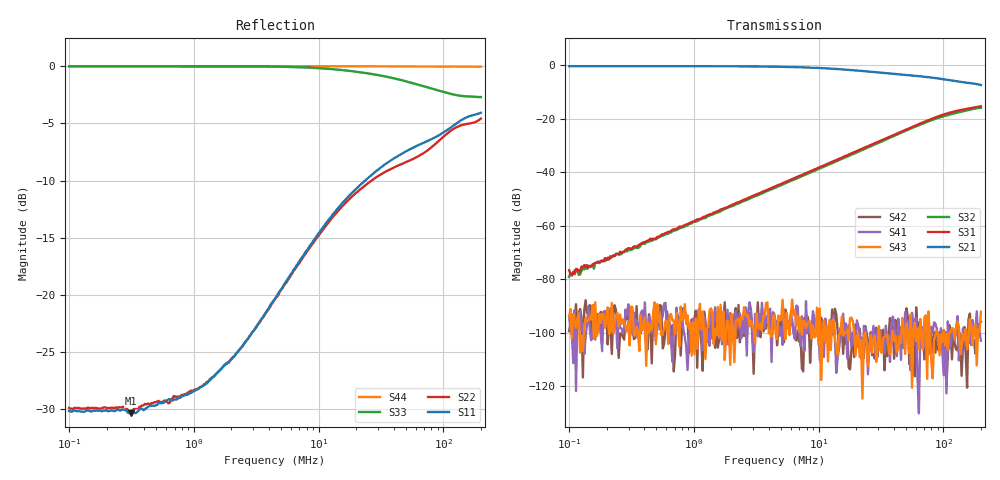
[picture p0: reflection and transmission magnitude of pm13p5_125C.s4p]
!Keysight Technologies,E5080A,MY55200740,A.12.60.03
!Date: Friday, October 02, 2020 16:46:49
!Correction: S11(Full 4 Port(1,2,3,4))
!S12(Full 4 Port(1,2,3,4))
!S13(Full 4 Port(1,2,3,4))
!S14(Full 4 Port(1,2,3,4))
!S21(Full 4 Port(1,2,3,4))
!S22(Full 4 Port(1,2,3,4))
!S23(Full 4 Port(1,2,3,4))
!S24(Full 4 Port(1,2,3,4))
!S31(Full 4 Port(1,2,3,4))
!S32(Full 4 Port(1,2,3,4))
!S33(Full 4 Port(1,2,3,4))
!S34(Full 4 Port(1,2,3,4))
!S41(Full 4 Port(1,2,3,4))
!S42(Full 4 Port(1,2,3,4))
!S43(Full 4 Port(1,2,3,4))
!S44(Full 4 Port(1,2,3,4))
!S4P File: Measurements: <S11,S12,S13,S14>,
!<S21,S22,S23,S24>,
!<S31,S32,S33,S34>,
!<S41,S42,S43,S44>:Log Frequency Sweep
# Hz S  dB  R 50
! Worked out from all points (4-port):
!   300 points, 100 kHz to 200 MHz, reference 50 ohm
!   strongest paths, dB at 100 kHz, 673 kHz, 4.529 MHz, 30.48 MHz, 200 MHz:
!     S21: -0.3, -0.3, -0.5, -2.6, -7.3
!     S31: -76.7, -61.5, -45.2, -28.4, -15.3
!     S32: -79.2, -62.0, -45.7, -28.9, -15.8
!     S43: -94.1, -95.5, -100.3, -97.6, -92.3
!     S41: -93.9, -111.0, -96.1, -104.5, -103.1
!     S42: -99.5, -97.3, -95.8, -100.9, -95.9
!   lowest |S11| = -30.3 dB at 313.9 kHz (marker M1), VSWR 1.06, Z = 53.1 - j0.415 ohm
!   |S11| at or under -10 dB: start of sweep to 23.56 MHz
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100000  -30.14 0.8  -0.28 -0.2  -77.77 103.0  -90.92 60.2
        -0.28 -0.1  -29.86 1.1  -78.88 67.9  -85.22 -115.2
        -76.69 78.8  -79.15 95.1  0.00 -0.1  -95.41 -79.3
        -93.87 -113.2  -99.46 -33.6  -94.12 -60.1  0.00 -0.0
105215.7  -30.20 0.5  -0.28 -0.2  -77.80 83.2  -103.98 -155.2
          -0.28 -0.1  -29.93 0.4  -80.37 91.0  -96.15 -156.7
          -78.67 102.4  -78.51 85.9  0.00 -0.1  -101.36 73.9
          -100.97 114.8  -98.27 -113.1  -102.19 69.2  0.00 -0.0
313913.9  -30.34 -7.4  -0.28 -0.4  -68.51 89.4  -97.13 -67.5
          -0.28 -0.4  -30.13 -7.3  -68.75 92.7  -117.84 -154.3
          -68.65 89.8  -69.02 84.8  0.00 -0.4  -93.11 13.3
          -92.06 -106.5  -98.51 -102.1  -90.35 37.1  0.00 -0.0
1908390  -25.91 -59.9  -0.31 -2.4  -52.70 89.4  -98.68 -167.1
         -0.32 -2.4  -25.81 -57.8  -53.15 89.7  -89.17 141.3
         -52.77 89.4  -53.09 89.8  -0.01 -2.3  -95.01 -3.0
         -104.70 148.2  -95.32 36.3  -97.84 -14.1  0.00 -0.1
2.13545e7  -10.42 -127.6  -1.98 -13.9  -31.53 84.7  -100.19 -137.0
           -1.99 -13.9  -10.81 -116.8  -32.07 87.7  -91.22 2.2
           -31.57 84.7  -32.08 87.7  -0.52 -22.9  -107.95 164.1
           -101.37 70.1  -98.53 103.7  -109.23 149.9  -0.00 -1.4
8.215269e7  -6.33 -150.0  -4.59 -15.6  -19.85 64.0  -98.02 -95.8
            -4.60 -15.6  -6.99 -128.3  -20.33 72.5  -99.33 34.0
            -19.85 63.9  -20.34 72.5  -1.97 -66.0  -101.85 -150.7
            -100.07 -43.7  -107.39 159.4  -117.21 -127.5  -0.02 -5.7
2e8  -4.06 -160.3  -7.32 -8.8  -15.29 30.6  -99.46 -129.5
     -7.33 -8.8  -4.57 -107.7  -15.84 54.0  -94.10 79.7
     -15.29 30.7  -15.84 54.1  -2.69 -110.1  -93.15 -126.9
     -103.07 -73.9  -95.90 86.4  -92.28 -95.9  -0.04 -13.4
